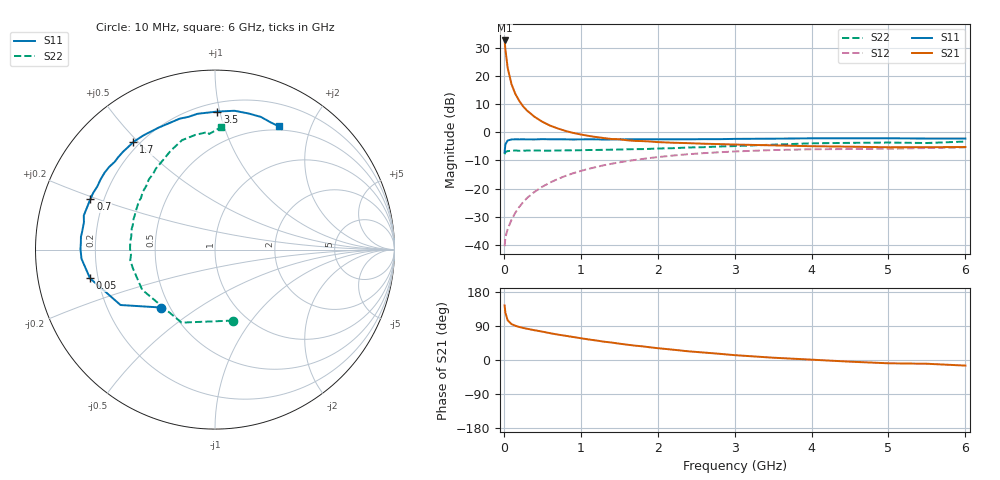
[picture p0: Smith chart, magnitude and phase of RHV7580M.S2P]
! SIEMENS Small Signal Semiconductors
! BFR106
! Si NPN RF Bipolar Junction Transistor in SOT23
! VCE = 0.75 V  IC = 80 mA
! Common Emitter S-Parameters:  August  1996
# GHz  S  MA  R  50
!  f  S11  S21  S12  S22
! GHz  MAG  ANG  MAG  ANG  MAG  ANG  MAG  ANG
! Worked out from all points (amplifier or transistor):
!   36 points, 10 MHz to 6 GHz, reference 50 ohm
!   highest |S21| = 32.5 dB at 10 MHz (marker M1)
!   |S21| within 3 dB of that: start of sweep to 19.61 MHz
!   unconditionally stable (mu >= 1): 54.98 MHz to end of sweep
!   at 250 MHz: K = 1.43, MAG = 13.1 dB, |S12| = -24.8 dB
!   at 1.4 GHz: K = 1.27, MAG = 1.3 dB, |S12| = -11.2 dB
!   at 6 GHz: K = 1.04, MAG = -1.1 dB, |S12| = -5.4 dB
!   S11 on the Smith chart (normalised r, x): 10 MHz: 0.45, -0.36; 50 MHz: 0.17, -0.11; 700 MHz: 0.15, +0.19; 1.7 GHz: 0.18, +0.48; 3.5 GHz: 0.26, +0.98; 6 GHz: 0.45, +1.55
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0.01  0.4399 -132.8  42.25 144.1  0.0096 55.8  0.408 -75.7
0.02  0.6102 -149.6  29.5 124.7  0.0136 46.3  0.4474 -114.6
0.05  0.7147 -167.1  13.72 104.6  0.0194 47.8  0.4634 -151.1
0.1  0.7456 -176.1  7.07 94.8  0.0282 58.0  0.4694 -167.3
0.15  0.7495 179.8  4.76 90.3  0.0377 63.1  0.4755 -172.9
0.2  0.7483 177.2  3.604 87.2  0.0475 66.4  0.469 -176.5
0.25  0.7503 174.5  2.879 84.6  0.0576 67.9  0.4724 -179.4
0.3  0.747 172.5  2.43 82.6  0.0682 69.5  0.4734 179.0
0.4  0.746 168.2  1.873 78.5  0.0881 69.5  0.4737 175.6
0.5  0.7554 165.4  1.536 74.9  0.1083 69.0  0.4733 172.9
0.6  0.7503 161.4  1.313 70.8  0.1284 67.9  0.4721 170.6
0.7  0.7494 157.9  1.169 67.1  0.1482 66.4  0.4759 168.4
0.9  0.7441 151.9  0.975 60.7  0.1876 62.8  0.4779 163.6
1.1  0.7498 145.1  0.863 54.3  0.2244 59.1  0.4846 159.7
1.7  0.752 127.4  0.703 38.0  0.3224 46.9  0.5022 147.1
2.2  0.7487 114.9  0.652 27.2  0.387 37.0  0.5218 137.2
3  0.763 97.3  0.606 12.8  0.4568 22.4  0.569 122.3
3.5  0.7692 89.0  0.586 6.1  0.4836 14.9  0.603 114.3
4.5  0.7811 76.1  0.555 -4.4  0.5048 1.7  0.6486 99.6
5  0.7822 70.9  0.542 -8.7  0.5103 -3.4  0.6564 93.4
5.5  0.7735 66.3  0.543 -9.9  0.5254 -5.9  0.6448 92.9
6  0.7734 62.7  0.548 -14.8  0.5395 -11.8  0.6841 87.0
